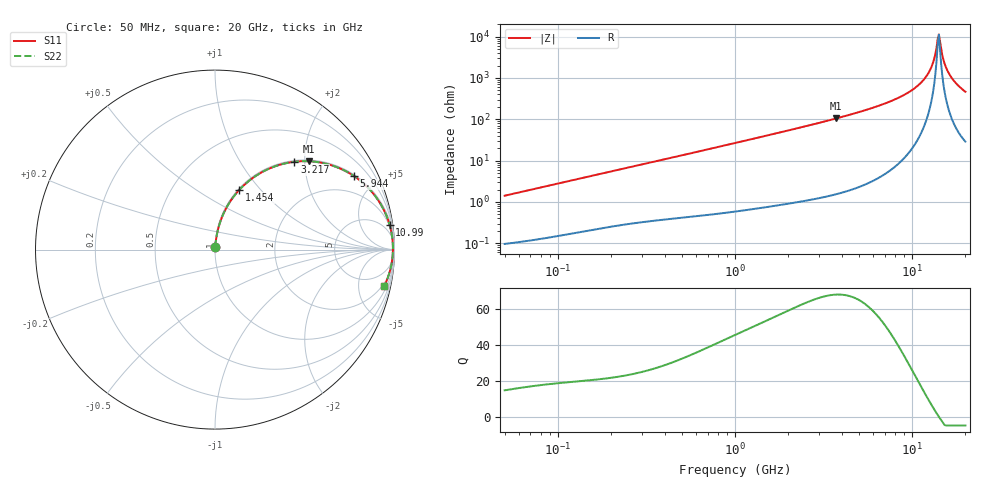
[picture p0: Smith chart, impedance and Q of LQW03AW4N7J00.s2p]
!Murata Part Number: LQW03AW4N7J00
!These Parameters are Measured in Series Mode Connection
!  o--[Z]--o
!Port1  Port2
!  o-------o
!Freq. Start=50[MHz] Stop=20[GHz], 401[Steps]
# Hz S RI R 50
!Freq.(Hz) S11(Real) S11(Imag) S21(Real) S21(Imag) S12(Real) S12(Imag) S22(Real) S22(Imag)
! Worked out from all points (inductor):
!   401 points, 50 MHz to 20 GHz, reference 50 ohm
!   read as one part in series: L = 4.48 nH near 51.52 MHz
!   highest Q = 68.1 at 3.736 GHz (marker M1), where L = 4.48 nH
!   self-resonance near 13.96 GHz
!   S11 on the Smith chart (normalised r, x): 50 MHz: 1.00, +0.03; 1.454 GHz: 1.01, +0.78; 3.217 GHz: 1.03, +1.78; 5.944 GHz: 1.06, +3.75; 10.99 GHz: 2, +14; 20 GHz: 1.58, -9.26
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5e7  0.00116 0.0141  0.9988 -0.0141  0.9988 -0.0141  0.00116 0.0141
1.364002e8  0.00331 0.0375  0.9967 -0.0375  0.9967 -0.0375  0.00331 0.0375
3.721004e8  0.0134 0.0984  0.9866 -0.0984  0.9866 -0.0984  0.0134 0.0984
1e9  0.071 0.2461  0.929 -0.2461  0.929 -0.2461  0.071 0.2461
1.454215e9  0.1356 0.333  0.8644 -0.333  0.8644 -0.333  0.1356 0.333
2.728004e9  0.3582 0.4719  0.6418 -0.4719  0.6418 -0.4719  0.3582 0.4719
3.216634e9  0.4423 0.4893  0.5577 -0.4893  0.5577 -0.4893  0.4423 0.4893
3.736399e9  0.5245 0.4921  0.4755 -0.4921  0.4755 -0.4921  0.5245 0.4921
5.944466e9  0.7749 0.4093  0.2251 -0.4093  0.2251 -0.4093  0.7749 0.4093
7.442007e9  0.8709 0.3249  0.1291 -0.3249  0.1291 -0.3249  0.8709 0.3249
9.316812e9  0.9404 0.2213  0.0596 -0.2213  0.0596 -0.2213  0.9404 0.2213
1.098561e10  0.973 0.1373  0.027 -0.1373  0.027 -0.1373  0.973 0.1373
1.183995e10  0.9825 0.0975  0.0175 -0.0975  0.0175 -0.0975  0.9825 0.0975
1.257102e10  0.9877 0.0651  0.0123 -0.0651  0.0123 -0.0651  0.9877 0.0651
1.314879e10  0.9901 0.0404  0.0099 -0.0404  0.0099 -0.0404  0.9901 0.0404
1.375312e10  0.9913 0.0155  0.00874 -0.0155  0.00874 -0.0155  0.9913 0.0155
1.417136e10  0.9913 -0.00127  0.00869 0.00127  0.00869 0.00127  0.9913 -0.00127
1.438523e10  0.9911 -0.00969  0.00889 0.00969  0.00889 0.00969  0.9911 -0.00969
1.527346e10  0.9888 -0.0436  0.0112 0.0436  0.0112 0.0436  0.9888 -0.0436
1.621653e10  0.984 -0.0779  0.016 0.0779  0.016 0.0779  0.984 -0.0779
1.774144e10  0.9716 -0.13  0.0284 0.13  0.0284 0.13  0.9716 -0.13
2e10  0.9443 -0.2004  0.0557 0.2004  0.0557 0.2004  0.9443 -0.2004
